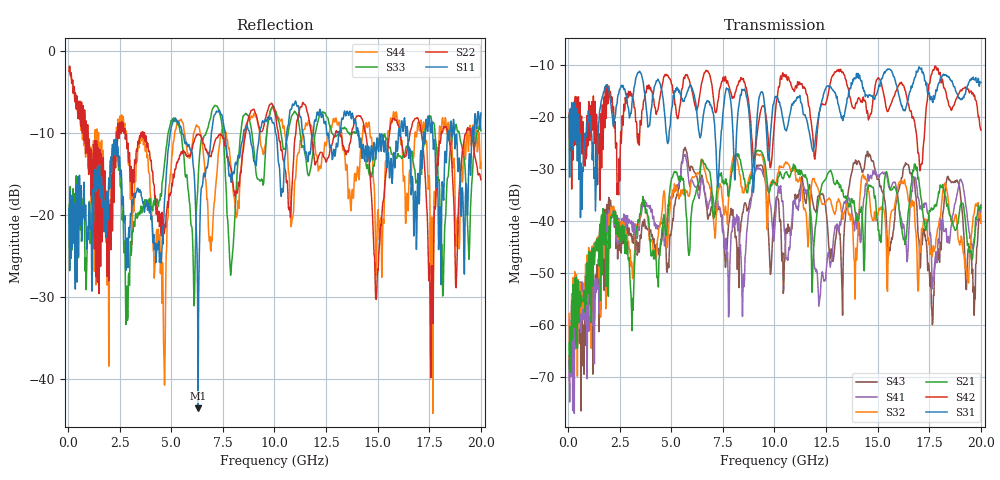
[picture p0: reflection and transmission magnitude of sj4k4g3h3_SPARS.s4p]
! FILE: E:\users\goganessyan\GBX_Backplane\FR408_backplane\1m_INBOUND_NEXT\sj4k4g3h3_SPARS.s4p
# MHZ S RI R 50.00
! FREQ  S11  S12  S13  S14
!  S21  S22  S23  S24
!  S31  S32  S33  S34
!  S41  S42  S43  S44
!  REAL  IMAG  REAL  IMAG  REAL  IMAG  REAL  IMAG
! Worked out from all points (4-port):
!   799 points, 50 MHz to 20 GHz, reference 50 ohm
!   strongest paths, dB at 50 MHz, 5.025 GHz, 10.03 GHz, 15.03 GHz, 20 GHz:
!     S31: -19.7, -18.2, -16.1, -14.7, -13.4
!     S42: -19.3, -13.8, -19.8, -12.4, -22.5
!     S21: -63.5, -31.6, -32.6, -41.8, -37.1
!     S32: -57.8, -34.9, -32.6, -38.5, -40.4
!     S41: -66.9, -35.8, -40.6, -31.1, -36.9
!     S43: -65.9, -41.4, -37.9, -32.0, -37.0
!   lowest |S11| = -43.6 dB at 6.3 GHz (marker M1), VSWR 1.01, Z = 49.9 - j0.655 ohm
!   |S11| at or under -10 dB: start of sweep to 4.948 GHz; 5.52 GHz to 6.947 GHz (1.427 GHz wide, 22.9 % of centre); 14.08 GHz to 16.01 GHz (1.932 GHz wide, 12.8 % of centre)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
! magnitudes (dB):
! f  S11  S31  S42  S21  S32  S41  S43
! 50 MHz  -19.2  -19.7  -19.3  -63.5  -57.8  -66.9  -65.9
! 2.025 GHz  -16.8  -16.2  -15.3  -45.2  -41.2  -41.5  -38.1
! 4.625 GHz  -21.5  -17.3  -12.4  -39.6  -34.8  -41.7  -39.2
! 6.3 GHz  -43.6  -21.6  -17.8  -32.8  -30.9  -35.0  -32.8
! 16.43 GHz  -9.2  -17.3  -16.5  -40.8  -34.2  -47.8  -29.1
! 17.65 GHz  -9.1  -17.0  -11.2  -37.9  -46.6  -53.0  -59.9
! 20 GHz  -7.6  -13.4  -22.5  -37.1  -40.4  -36.9  -37.0
